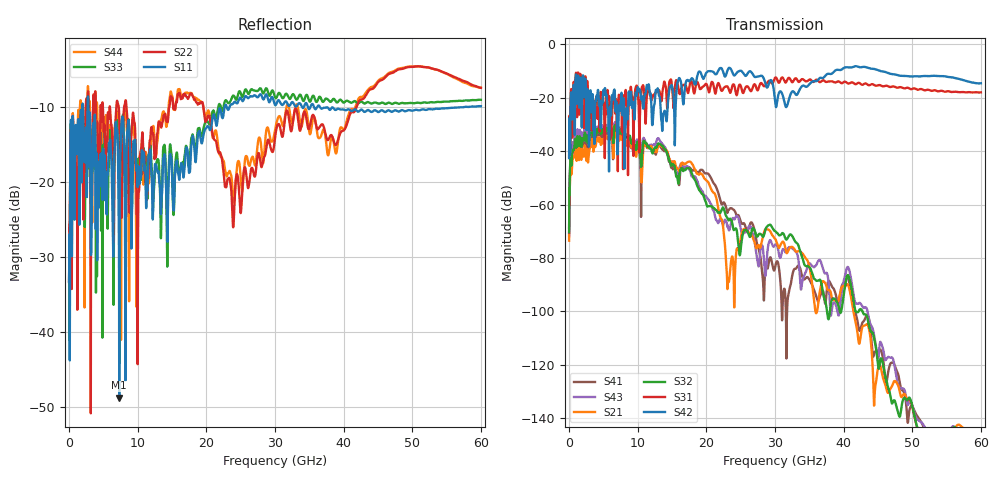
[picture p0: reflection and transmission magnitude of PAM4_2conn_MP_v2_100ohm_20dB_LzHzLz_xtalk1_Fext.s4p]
! Info: Touchstone file created by Circ.  Input file=FAB50GbE_2conn_Midplane_Examax_Topo2_v2_100ohm_20dB_LzHzLz.circ
# Hz S RI R 50
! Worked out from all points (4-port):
!   6000 points, 10 MHz to 60 GHz, reference 50 ohm
!   strongest paths, dB at 10 MHz, 15.01 GHz, 30.01 GHz, 45.01 GHz, 60 GHz:
!     S42: -42.6, -15.7, -21.2, -9.7, -14.6
!     S31: -42.2, -16.4, -12.6, -15.3, -18.0
!     S32: -70.4, -45.0, -69.9, -119.9, -153.0
!     S21: -73.5, -43.9, -72.8, -121.4, -147.8
!     S43: -71.6, -44.5, -75.0, -118.4, -153.0
!     S41: -68.7, -46.0, -83.7, -114.7, -150.9
!   lowest |S11| = -48.8 dB at 7.31 GHz (marker M1), VSWR 1.01, Z = 50.1 + j0.354 ohm
!   |S11| at or under -10 dB: start of sweep to 1.939 GHz; 2.806 GHz to 22.67 GHz (19.86 GHz wide, 156 % of centre); 36.57 GHz to 57.4 GHz (20.83 GHz wide, 44.3 % of centre)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
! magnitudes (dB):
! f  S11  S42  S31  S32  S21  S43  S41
! 10 MHz  -33.3  -42.6  -42.2  -70.4  -73.5  -71.6  -68.7
! 1.07 GHz  -14.2  -12.6  -11.8  -38.2  -42.1  -35.6  -38.2
! 7.31 GHz  -48.8  -22.9  -19.9  -33.3  -36.1  -32.1  -34.8
! 19.38 GHz  -14.7  -12.0  -16.1  -56.1  -48.7  -54.9  -47.0
! 23.14 GHz  -10.3  -9.4  -16.1  -65.3  -87.8  -68.0  -62.4
! 28.2 GHz  -8.8  -12.1  -15.1  -71.9  -72.6  -75.8  -87.2
! 60 GHz  -9.9  -14.6  -18.0  -153.0  -147.8  -153.0  -150.9
